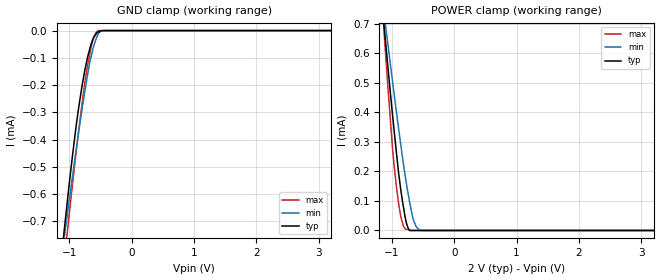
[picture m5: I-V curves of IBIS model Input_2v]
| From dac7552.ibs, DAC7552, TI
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|   Model   - Input_2V
[Model]   Input_2v
Model_type   Input
Vinl = 0
Vinh = 2
|   typ   min   max
|   (nom PVT)   (Fast PVT)   (slow PVT)
|Average
C_comp   1.885e-13   1.670e-13   2.024e-13
| Where   nom  PVT is  Nominal Process, 2.0V, 25C
|   Fast PVT is Strong Process, 2.2V, -40C
|   Slow PVT is Weak Process, 1.8V, 105C
[Voltage Range]   2   1.8   2.2
|Ambient Temperature   25   105   -40
|Junction Temperature
[Temperature Range]   25   105   -40
[Power Clamp Reference]   2   1.8   2.2
[GND Clamp Reference]   0   0   0
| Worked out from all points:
|   GND clamp passes 1 mA (typ) near -1.20 V on its own axis
|   POWER clamp passes 1 mA (typ) near -1.26 V on its own axis
[GND Clamp]
|   Voltage   I(typ)   I(min)   I(max)
-2V       -2.903mA   -2.411mA   -3.739mA
-1.092V   -752.6uA   -776.5uA   -875.9uA
-1.041V   -643.2uA   -688.4uA   -756.7uA
-1.012V   -581.7uA   -638.8uA   -694.2uA
-892mV    -350.8uA   -438.6uA   -446.9uA
-794mV    -198.9uA   -283.3uA   -264.1uA
-730.6mV  -122.3uA   -192.7uA   -158.8uA
-662.4mV  -58.39uA   -106.1uA   -72.88uA
-609.6mV  -25.15uA   -56.94uA   -25.28uA
-550.2mV  -6.981uA   -19.3uA    -1.858uA
-464.6mV  0A         0A         0A
4V        0A         0A         0A
[POWER Clamp]
|   Voltage   I(typ)   I(min)   I(max)
-2V       2.788mA    2.31mA     3.599mA
-1.149V   745.8uA    776uA      744.6uA
-1.112V   661.8uA    712.6uA    630.1uA
-1.102V   640.4uA    696.1uA    600.8uA
-988mV    388.2uA    501.7uA    273.8uA
-922mV    253.3uA    392.6uA    139.7uA
-856mV    136.3uA    288.5uA    46.39uA
-779mV    37.14uA    174.8uA    3.903uA
-732mV    4.481uA    116.1uA    2.482uA
-650mV    0A         33.84uA    0A
-530mV    0A         82.34nA    0A
4V        0A         0A         0A
